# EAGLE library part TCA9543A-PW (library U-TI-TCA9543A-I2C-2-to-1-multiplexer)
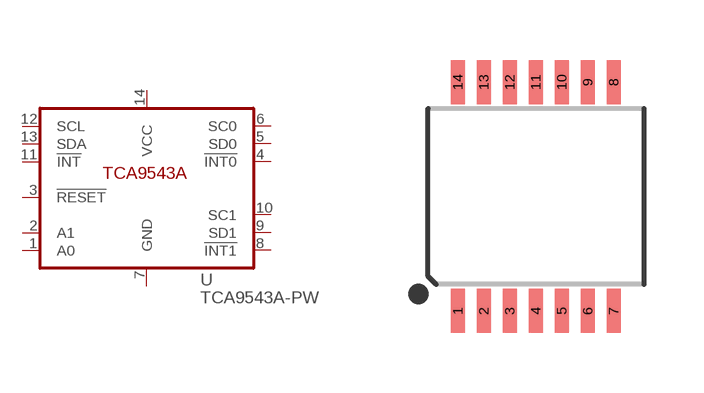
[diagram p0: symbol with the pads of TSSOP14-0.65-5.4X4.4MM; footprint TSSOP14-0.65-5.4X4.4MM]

Designator prefix U

## TCA9543A-PW  [TSSOP14-0.65-5.4X4.4MM]
1  A0  in
2  A1  in
3  !RESET  in
4  !INT0  in
5  SD0
6  SC0  out
7  GND  pwr
8  !INT1  in
9  SD1
10  SC1  out
11  !INT  oc
12  SCL  in
13  SDA
14  VCC  pwr

## Footprint TSSOP14-0.65-5.4X4.4MM (pad centres in mm)
TSSOP-14
smd 0.35 x 1.1: 1 -1.95,-2.86; 2 -1.3,-2.86; 3 -0.65,-2.86; 4 0,-2.86; 5 0.65,-2.86; 6 1.3,-2.86; 7 1.95,-2.86; 8 1.95,2.86; 9 1.3,2.86; 10 0.65,2.86; 11 0,2.86; 12 -0.65,2.86; 13 -1.3,2.86; 14 -1.95,2.86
